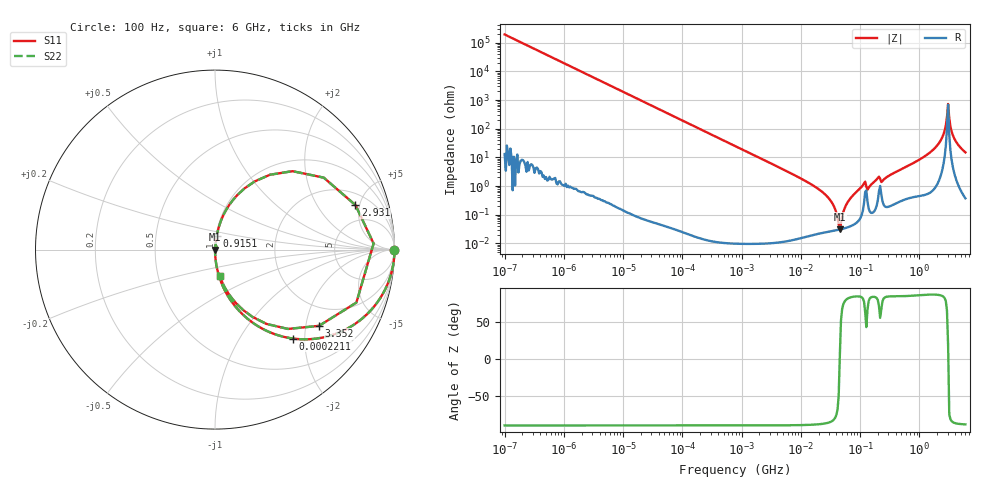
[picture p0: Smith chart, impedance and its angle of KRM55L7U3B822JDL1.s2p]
!Murata Part Number: KRM55L7U3B822JDL1
!These Parameters are Measured in Series Mode Connection
!Data Generated on Jan 08, 2026
!  o--ll--o
!Port1  Port2
!  o------o
!Operation Temp=25[degC], DC Bias Voltage=0[V]
!Freq. Start=100[Hz] Stop=6[GHz] 401[Steps]
# Hz S RI R 50
!Freq.(Hz) S11(Real) S11(Imag) S21(Real) S21(Imag) S12(Real) S12(Imag) S22(Real) S22(Imag)
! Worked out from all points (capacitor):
!   401 points, 100 Hz to 6 GHz, reference 50 ohm
!   read as one part in series: C = 8.19 nF near 109 Hz
!   lowest |Z| = 30.6 mohm at 45.56 MHz (marker M1)
!   series resonance near 45.43 MHz, so ESL is about 1.5 nH
!   S11 on the Smith chart (normalised r, x): 100 Hz: open; 221.1 kHz: 1.00, -1.76; 915.1 MHz: 1.01, +0.15; 2.931 GHz: 3.00, +4.56; 3.352 GHz: 1.35, -2.38; 6 GHz: 1.01, -0.30
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100  1 -0.000515  3e-07 0.000515  3e-07 0.000515  1 -0.000515
2008  0.9999 -0.0103  0.000108 0.0103  0.000108 0.0103  0.9999 -0.0103
40335  0.9586 -0.1991  0.0414 0.1991  0.0414 0.1991  0.9586 -0.1991
94437  0.8088 -0.3932  0.1912 0.3932  0.1912 0.3932  0.8088 -0.3932
221108  0.4356 -0.4958  0.5644 0.4958  0.5644 0.4958  0.4356 -0.4958
774597  0.0592 -0.2358  0.9408 0.2358  0.9408 0.2358  0.0592 -0.2358
1.555665e7  0.000313 -0.011  0.9997 0.011  0.9997 0.011  0.000313 -0.011
3.045065e7  0.00027 -0.00349  0.9997 0.00349  0.9997 0.00349  0.00027 -0.00349
4.556224e7  0.000305 2.44e-05  0.9997 -2.44e-05  0.9997 -2.44e-05  0.000305 2.44e-05
6.233367e7  0.000374 0.00278  0.9996 -0.00278  0.9996 -0.00278  0.000374 0.00278
1.115611e8  0.0015 0.0105  0.9985 -0.0105  0.9985 -0.0105  0.0015 0.0105
1.395531e8  0.00174 0.0085  0.9983 -0.0085  0.9983 -0.0085  0.00174 0.0085
1.909225e8  0.00235 0.0168  0.9976 -0.0168  0.9976 -0.0168  0.00235 0.0168
3.124326e8  0.00247 0.0232  0.9975 -0.0232  0.9975 -0.0232  0.00247 0.0232
9.150511e8  0.0098 0.0736  0.9902 -0.0736  0.9902 -0.0736  0.0098 0.0736
2.142435e9  0.1 0.2764  0.9 -0.2764  0.9 -0.2764  0.1 0.2764
2.562649e9  0.3062 0.4171  0.6938 -0.4171  0.6938 -0.4171  0.3062 0.4171
2.931063e9  0.7827 0.248  0.2173 -0.248  0.2173 -0.248  0.7827 0.248
3.352442e9  0.5794 -0.4248  0.4206 0.4248  0.4206 0.4248  0.5794 -0.4248
3.666503e9  0.2869 -0.4141  0.7131 0.4141  0.7131 0.4141  0.2869 -0.4141
4.009986e9  0.1551 -0.3353  0.8449 0.3353  0.8449 0.3353  0.1551 -0.3353
6e9  0.0254 -0.1453  0.9746 0.1453  0.9746 0.1453  0.0254 -0.1453
